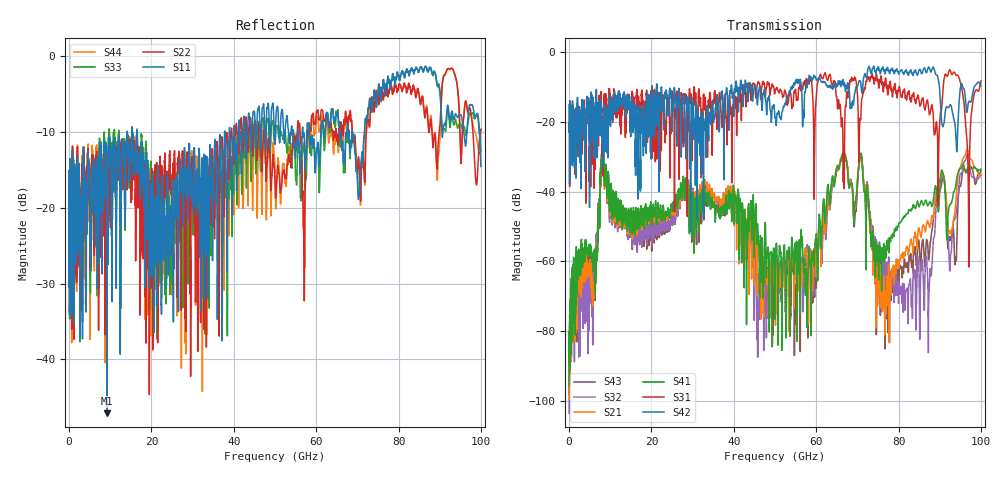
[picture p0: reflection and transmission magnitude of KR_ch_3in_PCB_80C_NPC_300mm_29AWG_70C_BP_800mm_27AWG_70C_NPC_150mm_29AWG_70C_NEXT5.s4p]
# Hz S RI R 45
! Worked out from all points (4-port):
!   4000 points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, 25 MHz to 100 GHz, reference 45 ohm
!   strongest paths, dB at 25 MHz, 25.02 GHz, 50.02 GHz, 75.03 GHz, 100 GHz:
!     S42: -20.7, -20.7, -18.8, -4.2, -9.7
!     S31: -20.7, -11.6, -11.3, -8.1, -8.3
!     S41: -95.8, -45.0, -71.0, -58.5, -33.6
!     S21: -99.5, -45.9, -65.8, -62.1, -35.0
!     S32: -103.7, -48.1, -70.0, -57.4, -35.3
!     S43: -98.3, -48.8, -70.7, -62.1, -34.1
!   lowest |S11| = -47.1 dB at 9.225 GHz (marker M1), VSWR 1.01, Z = 45.2 + j0.365 ohm
!   |S11| at or under -10 dB: start of sweep to 14.12 GHz; 16.48 GHz to 37.77 GHz (21.29 GHz wide, 78.5 % of centre); 68.84 GHz to 71.74 GHz (2.899 GHz wide, 4.12 % of centre)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
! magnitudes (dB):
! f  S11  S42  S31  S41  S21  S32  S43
! 25 MHz  -16.4  -20.7  -20.7  -95.8  -99.5  -103.7  -98.3
! 9.225 GHz  -47.1  -28.9  -24.4  -38.1  -39.3  -40.2  -39.1
! 49.73 GHz  -8.3  -15.1  -10.1  -56.4  -57.0  -62.7  -62.8
! 70.78 GHz  -15.0  -8.4  -19.4  -29.1  -30.0  -29.6  -29.1
! 76.58 GHz  -4.1  -5.2  -9.0  -58.8  -67.7  -60.7  -64.7
! 96.9 GHz  -7.9  -14.9  -35.3  -33.1  -28.7  -29.1  -34.3
! 100 GHz  -14.6  -9.7  -8.3  -33.6  -35.0  -35.3  -34.1
